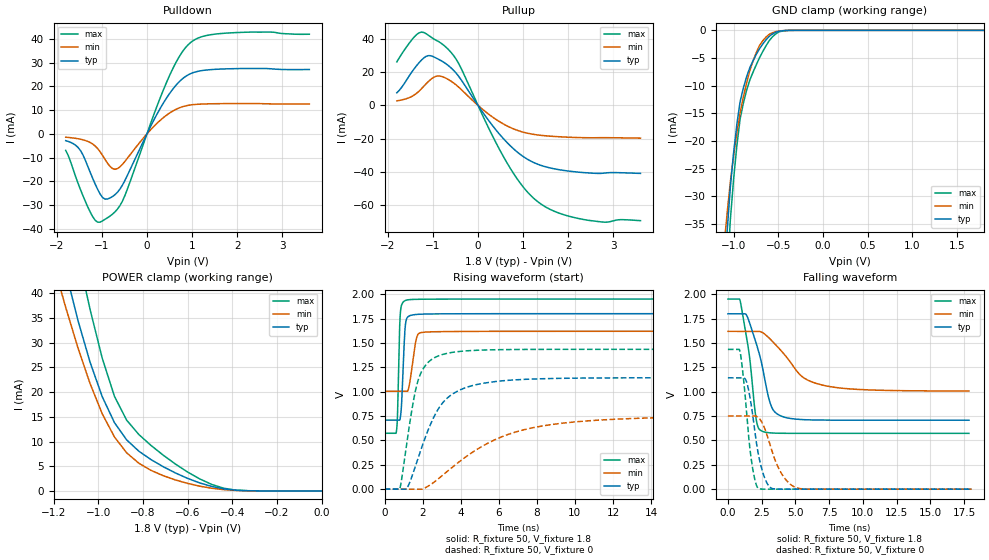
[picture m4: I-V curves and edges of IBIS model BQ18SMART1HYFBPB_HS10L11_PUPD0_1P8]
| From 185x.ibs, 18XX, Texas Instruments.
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|   Model Cell BQ18SMART1HYFBPB_HS10L11_PUPD0_1P8
|BQ18SMART1HYFBPB_HS10L11_PUPD0_1P8
[Model]   BQ18SMART1HYFBPB_HS10L11_PUPD0_1P8
Model_type   I/O
Polarity   Non-Inverting
Enable   Active-Low
Vinl =  0.63
Vinh =  1.17
Cref =  15pF
Rref =  100.0000M
Vref =  0V
Vmeas =  0.9
C_comp   0.915143p   0.8088923p   1.028577p
[Model Spec]
Vinl   0.63   0.567   0.6825
Vinh   1.17   1.053   1.2675
[Temperature Range]   25   125   -40
[Voltage Range]   1.8   1.62   1.95
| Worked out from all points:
|   slope of the pulldown table from 0 to 0.27 V, typ, clamps not added: 27.2 ohm
|   slope of the pullup table from 0 to 0.27 V, typ, clamps not added: 26 ohm
|   GND clamp passes 1 mA (typ) near -0.59 V on its own axis
|   POWER clamp passes 1 mA (typ) near -0.50 V on its own axis
|   rising waveform, R_fixture 50, V_fixture 1.8: 20-80 % time 146ps typ, 269ps min, 101ps max; typ from 0.708 V to 1.8 V
|   rising waveform, R_fixture 50, V_fixture 0: 20-80 % time 1.58ns typ, 3.94ns min, 782ps max; typ from 0 V to 1.14 V
|   falling waveform, R_fixture 50, V_fixture 1.8: 20-80 % time 1.14ns typ, 2.34ns min, 734ps max; typ from 1.8 V to 0.708 V
|   falling waveform, R_fixture 50, V_fixture 0: 20-80 % time 797ps typ, 1.23ns min, 606ps max; typ from 1.14 V to 0 V
| Nom Voltages:
|   BIASFET=1.8, VBBNW=1.1, VDD=1.1, VDDS=1.8, VSS=0, VSSS=0
| Min Voltages:
|   BIASFET=1.62, VBBNW=0.99, VDD=0.99, VDDS=1.62, VSS=0, VSSS=0
| Max Voltages:
|   BIASFET=1.95, VBBNW=1.21, VDD=1.21, VDDS=1.95, VSS=0, VSSS=0
[POWER_clamp]
|   voltage   I(typ)   I(min)   I(max)
-1.8V     196.8mA    157.5mA    250.4mA
-1.164V   48mA       40.06mA    64.23mA
-1.127V   41.11mA    34.43mA    55.95mA
-1.109V   37.83mA    31.72mA    51.94mA
-1.055V   28.88mA    24.15mA    40.47mA
-981.8mV  19.06mA    15.6mA     26.85mA
-927.3mV  13.83mA    10.93mA    19.15mA
-872.7mV  10.34mA    7.72mA     14.33mA
-763.6mV  6.344mA    4.165mA    9.211mA
-600mV    2.546mA    1.527mA    3.832mA
-436.4mV  402.5uA    253uA      527.5uA
0V        291.8pA    1.073nA    4.224nA
[Pulldown]
|   voltage   I(typ)   I(min)   I(max)
-1.8V     -2.835mA   -1.376mA   -6.938mA
-1.473V   -6.994mA   -2.229mA   -23.44mA
-1.2V     -18.79mA   -4.282mA   -34.89mA
-1.036V   -25.33mA   -7.531mA   -37.14mA
-872.7mV  -27.39mA   -12.36mA   -35.28mA
-654.5mV  -24.59mA   -14.63mA   -31.68mA
-490.9mV  -19.69mA   -11.65mA   -26.08mA
381.8mV   13.54mA    7.117mA    19.32mA
654.5mV   20.72mA    10.44mA    30.48mA
927.3mV   25mA       12.07mA    37.79mA
1.636V    27.3mA     12.74mA    42.26mA
3.6V      27.12mA    12.64mA    41.97mA
[Pullup]
|   voltage   I(typ)   I(min)   I(max)
-1.8V     7.614mA    2.74mA     26.22mA
-1.527V   17.69mA    4.626mA    37.43mA
-1.309V   25.69mA    8.541mA    43.72mA
-1.036V   29.87mA    15.94mA    41.05mA
-818.2mV  26.95mA    17.52mA    37.49mA
-490.9mV  19.61mA    12.45mA    28.08mA
545.5mV   -19.54mA   -10.94mA   -30.03mA
927.3mV   -29.38mA   -15.56mA   -46.58mA
1.255V    -34.7mA    -17.56mA   -56.51mA
1.691V    -38.25mA   -18.74mA   -63.85mA
2.291V    -40.42mA   -19.45mA   -68.55mA
3.6V      -41.01mA   -19.75mA   -69.5mA
[GND_clamp]
|   voltage   I(typ)   I(min)   I(max)
-1.8V     -274mA     -200.4mA   -365.5mA
-1.109V   -45.37mA   -39.32mA   -55.85mA
-1.073V   -36.45mA   -33.1mA    -44.39mA
-1.036V   -28.3mA    -27.35mA   -34.22mA
-1V       -22.14mA   -22.69mA   -26.92mA
-927.3mV  -12.91mA   -14.91mA   -16.03mA
-854.5mV  -8.387mA   -9.532mA   -10.83mA
-781.8mV  -5.484mA   -5.512mA   -7.535mA
-709.1mV  -3.298mA   -2.71mA    -4.931mA
-600mV    -1.058mA   -705.2uA   -1.831mA
-381.8mV  -13.32uA   -12.31uA   -19.39uA
1.8V      291.8pA    820.3nA    4.087nA
[Ramp]
| variable   typ   min   max
dV/dt_f 0.65709767/1.1436036n 0.36978865/2.356738n  0.82844212/0.73686242n
dV/dt_r 0.69689023/1.5845599n 0.45844807/4.0755852n 0.87059979/0.78497193n
R_load = 50
[Rising Waveform]
R_fixture = 50
V_fixture = 1.8
V_fixture_min = 1.62
V_fixture_max = 1.95
|   time   V(typ)   V(min)   V(max)
0s        708.3mV    1.005V     573.3mV
619.2ps   708.3mV    1.005V     591.1mV
679ps     708.3mV    1.005V     779.6mV
775ps     708.3mV    1.005V     1.575V
822.2ps   731.1mV    1.005V     1.798V
1.114ns   1.717V     1.005V     1.937V
1.286ns   1.775V     1.056V     1.944V
1.677ns   1.792V     1.551V     1.947V
1.924ns   1.795V     1.607V     1.948V
17.87ns   1.8V       1.62V      1.95V
[Rising Waveform]
R_fixture = 50
V_fixture = 0
V_fixture_min = 0
V_fixture_max = 0
|   time   V(typ)   V(min)   V(max)
0s        0V         0V         0V
794.4ps   0V         0V         0V
1.149ns   0V         0V         449.7mV
1.477ns   153.9mV    0V         865.7mV
1.733ns   303.9mV    0V         1.099V
2.168ns   547.4mV    17.91mV    1.275V
2.81ns    819.8mV    104.5mV    1.366V
4.337ns   1.047V     341.5mV    1.419V
7.592ns   1.128V     622mV      1.434V
18.06ns   1.143V     743mV      1.434V
[Falling Waveform]
R_fixture = 50
V_fixture = 1.8
V_fixture_min = 1.62
V_fixture_max = 1.95
|   time   V(typ)   V(min)   V(max)
0s        1.8V       1.619V     1.95V
909.8ps   1.8V       1.619V     1.932V
1.578ns   1.718V     1.619V     1.385V
2.082ns   1.503V     1.619V     729.2mV
2.472ns   1.308V     1.613V     599.7mV
3.239ns   843.6mV    1.525V     576.5mV
4.21ns    737.5mV    1.378V     573mV
5.573ns   713.3mV    1.147V     572.6mV
7.303ns   708.4mV    1.059V     572.6mV
17.87ns   707.6mV    1.007V     572.6mV
[Falling Waveform]
R_fixture = 50
V_fixture = 0
V_fixture_min = 0
V_fixture_max = 0
|   time   V(typ)   V(min)   V(max)
0s        1.142V     751.5mV    1.434V
903.4ps   1.142V     751.5mV    1.409V
1.346ns   1.115V     751.5mV    853.1mV
1.711ns   880mV      751.5mV    326.7mV
2.002ns   587.1mV    751.5mV    94.15mV
2.256ns   359.5mV    734.1mV    7.203mV
3.098ns   22.5mV     465.6mV    0V
3.996ns   0V         155.1mV    0V
5.046ns   0V         15.96mV    0V
18.06ns   0V         0V         0V
